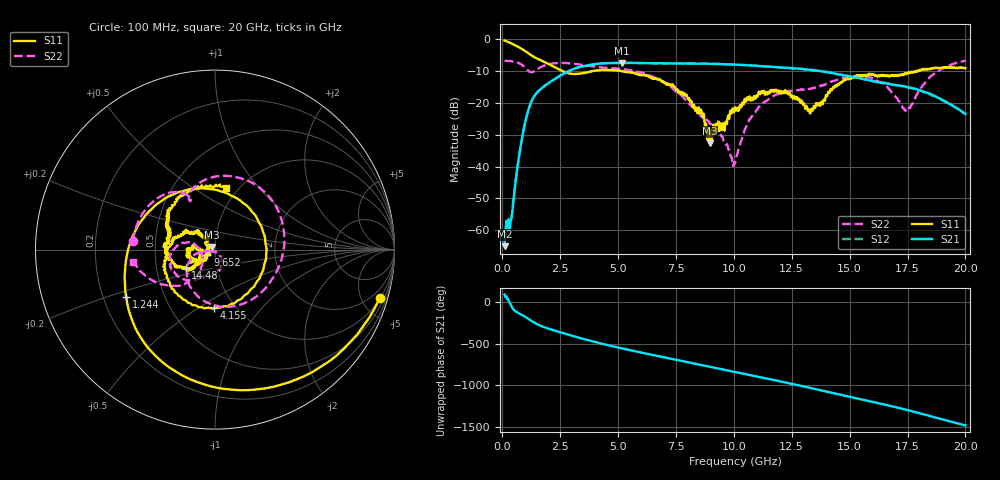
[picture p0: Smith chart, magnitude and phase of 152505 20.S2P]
!  2-Port S-parameters saved by WinCal
! VAR MeasName=S-Parameters (CALIBRATED_DATA) read from VNA (N5230C)
! VAR MeasDate=4/10/2015 9:30:16 AM
! VAR NAME=152505 20
! VAR FILENAME=152505 20.S2P
! VAR DATE=4/10/2015 9:30:16 AM
! VAR PHYS_PORTS=1,2
# Hz S DB R 50
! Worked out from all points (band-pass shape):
!   801 points, 100 MHz to 20 GHz, reference 50 ohm
!   highest |S21| = -7.41 dB at 5.15 GHz (marker M1); lowest = -65.0 dB at 100 MHz (marker M2)
!   |S21| within 3 dB of the highest: 2.747 GHz to 14.07 GHz (11.32 GHz wide, 135 % of centre)
!   lowest |S11| = -32.7 dB at 8.956 GHz (marker M3), VSWR 1.05, Z = 48.2 + j1.39 ohm
!   |S11| at or under -10 dB: 2.599 GHz to 3.871 GHz (1.272 GHz wide, 39.3 % of centre); 5.127 GHz to 17.88 GHz (12.75 GHz wide, 111 % of centre); 17.90871 GHz to 17.95199 GHz (43.28 MHz wide, 0.241 % of centre)
!   |S22| runs from -39.8 to -6.7 dB; largest |S21 - S12| = 0.0062
!   S11 on the Smith chart (normalised r, x): 100 MHz: 1.05, -6.79; 1.244 GHz: 0.30, -0.23; 4.155 GHz: 0.80, -0.58; 9.652 GHz: 0.92, -0.05; 14.48 GHz: 0.70, -0.15; 20 GHz: 0.88, +0.69
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1e8  -0.38 -16.4  -64.98 90.6  -63.72 68.5  -6.76 173.9
3.985e8  -1.36 -57.5  -56.02 -54.5  -55.83 -55.3  -6.91 155.2
5.72625e8  -1.97 -79.5  -44.73 -111.5  -44.68 -111.5  -7.15 144.0
8.96e8  -3.28 -117.0  -29.37 -163.2  -29.34 -163.1  -8.29 123.4
1.24425e9  -5.02 -151.9  -19.76 135.0  -19.72 134.9  -10.37 116.6
2.313875e9  -8.96 108.1  -12.24 11.9  -12.24 11.7  -7.51 72.6
3.43325e9  -10.73 -28.3  -8.55 -78.5  -8.56 -78.4  -8.05 13.6
4.154625e9  -9.74 -91.1  -7.69 -131.2  -7.68 -131.2  -8.74 -18.2
5.149625e9  -10.11 -143.6  -7.41 163.1  -7.43 163.1  -9.32 -59.7
6.741625e9  -12.37 163.6  -7.55 68.8  -7.53 68.4  -12.53 -129.5
7.861e9  -16.89 132.2  -7.63 4.9  -7.59 5.1  -18.59 -166.1
8.9555e9  -32.74 141.5  -7.73 -57.6  -7.74 -57.5  -26.49 -170.8
9.652e9  -25.83 -144.9  -7.89 -97.5  -7.87 -97.6  -33.09 -159.8
1.005e10  -21.40 -138.5  -7.97 -120.8  -7.97 -120.9  -39.03 -80.5
1.116938e10  -16.54 -156.7  -8.45 174.3  -8.38 174.2  -20.48 -64.3
1.236338e10  -17.34 179.6  -8.98 103.9  -9.08 103.7  -16.23 -101.7
1.338325e10  -22.32 -167.3  -9.69 41.4  -9.66 41.6  -15.30 -116.1
1.447775e10  -14.25 -147.6  -10.93 -27.6  -10.90 -27.7  -12.67 -132.8
1.669162e10  -11.63 164.8  -13.99 -166.0  -14.05 -167.2  -15.59 166.4
1.748762e10  -10.51 154.9  -15.02 139.9  -15.03 139.4  -22.36 -156.1
1.853238e10  -9.20 130.4  -17.32 63.6  -17.57 63.2  -11.49 -132.6
2e10  -9.13 79.5  -23.47 -45.3  -23.53 -44.6  -6.70 -171.2
